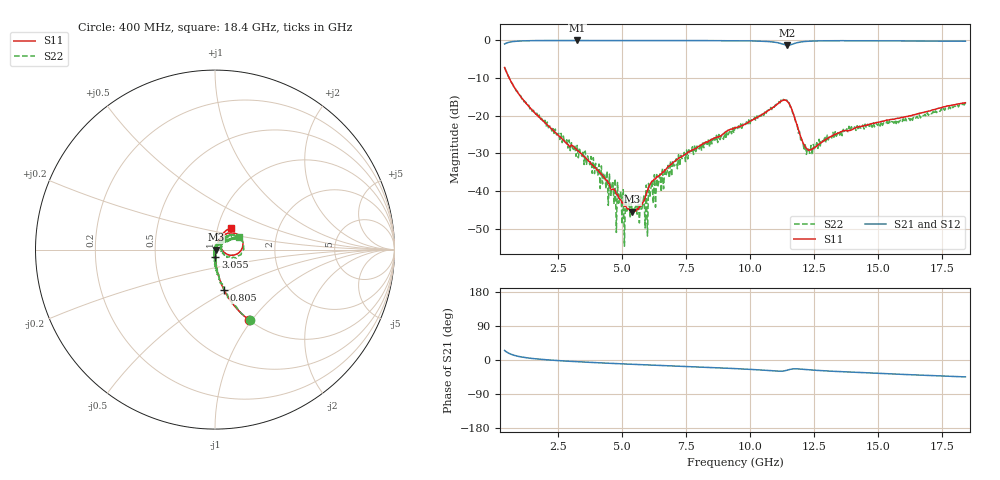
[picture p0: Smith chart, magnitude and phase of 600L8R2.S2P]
!  American Technical Ceramics  Date:  10/27/06
!  One Norden Lane
!  Huntington Station,  NY.  11746-2102
!  Tel:  (631) 622-4700  Fax:  (631) 622-4748
!  Part Number  600L8R2		Mounting Orientation: Vertical
!  Description: Ultra Low ESR Microwave capacitors
!  Application: Coupling, Bypass, Tuning, DC Block
!  Filters, Matching
# GHZ S DB R 50
! Freq  |S11|  S11 Ph  |S21|  S21 Ph  |S12|  S12 Ph  |S22|  S22 Ph
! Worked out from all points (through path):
!   401 points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, 400 MHz to 18.4 GHz, reference 50 ohm
!   highest |S21| = -0.04 dB at 3.235 GHz (marker M1); lowest = -1.3 dB at 11.43 GHz (marker M2)
!   group delay of S21, straight-line fit = 7.79 ps
!   lowest |S11| = -45.5 dB at 5.395 GHz (marker M3), VSWR 1.01, Z = 50.5 - j0.0848 ohm
!   |S11| at or under -10 dB: 577.2 MHz to end of sweep
!   |S22| runs from -54.7 to -7.1 dB; largest |S21 - S12| = 0.0063
!   S11 on the Smith chart (normalised r, x): 400 MHz: 1.00, -0.97; 805 MHz: 0.99, -0.47; 3.055 GHz: 1.00, -0.08; 18.4 GHz: 1.16, +0.28
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0.4  -7.23 -64.3  -0.98 25.1  -0.97 24.9  -7.14 -63.3
0.805  -12.77 -77.4  -0.28 11.8  -0.26 11.8  -12.54 -77.0
3.055  -28.03 -87.2  -0.05 -3.9  -0.03 -4.0  -28.72 -82.7
3.235  -29.20 -87.6  -0.04 -4.6  -0.03 -4.7  -27.91 -92.4
3.415  -30.21 -88.1  -0.05 -5.2  -0.03 -5.2  -30.78 -104.7
4.315  -36.73 -78.5  -0.05 -8.1  -0.03 -8.3  -35.69 -78.0
4.765  -40.92 -67.2  -0.05 -9.5  -0.04 -9.6  -51.02 -83.3
4.945  -42.39 -55.4  -0.05 -10.0  -0.04 -10.2  -40.12 -69.1
5.08  -44.08 -44.2  -0.05 -10.4  -0.04 -10.6  -54.67 28.1
5.215  -44.83 -32.9  -0.06 -10.8  -0.05 -11.0  -44.15 -169.9
5.395  -45.49 -9.1  -0.06 -11.3  -0.05 -11.5  -46.11 58.5
5.89  -41.85 45.7  -0.07 -12.7  -0.07 -12.9  -49.85 9.1
6.115  -37.88 49.3  -0.06 -13.3  -0.06 -13.5  -39.35 47.1
6.43  -35.95 51.3  -0.06 -14.2  -0.06 -14.4  -37.14 50.2
7.735  -29.06 60.0  -0.06 -17.9  -0.07 -18.1  -28.27 67.5
9.4  -23.31 62.1  -0.11 -22.7  -0.14 -23.0  -23.07 48.9
11.425  -16.10 7.9  -1.28 -27.1  -1.28 -27.2  -15.89 0.4
12.1  -27.83 -4.4  -0.33 -24.8  -0.35 -24.9  -29.23 -17.8
12.415  -28.91 29.7  -0.20 -26.5  -0.21 -26.6  -30.41 24.7
13.855  -23.95 61.2  -0.13 -31.9  -0.14 -31.9  -22.84 46.9
15.43  -21.12 63.0  -0.14 -36.5  -0.16 -36.5  -21.35 35.8
18.4  -16.58 53.0  -0.24 -44.6  -0.27 -44.5  -16.52 27.5
